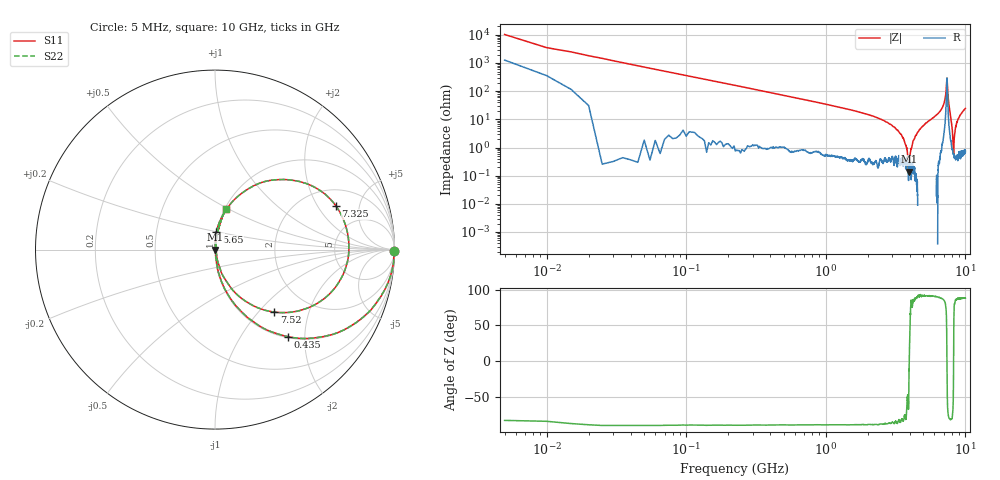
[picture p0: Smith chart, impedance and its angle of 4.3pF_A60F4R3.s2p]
! Amotech Co.,Ltd.
! http://www.amotech.co.kr/
! Part Number: A60F4R3
! These Parameters are Measured in Series Mode Connection
! Operation Temp=25[degC], DC Bias Voltage=0[V]
! Freq. Start=5[MHz] Stop=10[GHz], 2000[Steps]
! Date: Monday, July 20, 2020, 03:25:52
# GHZ S RI R 50.000000
!Freq.(Hz) S11(Real) S11(Imag) S21(Real) S21(Imag) S12(Real) S12(Imag) S22(Real) S22(Imag)
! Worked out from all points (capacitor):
!   2000 points, 5 MHz to 10 GHz, reference 50 ohm
!   read as one part in series: C = 4.43 pF near 55 MHz
!   lowest |Z| = 139 mohm at 3.935 GHz (marker M1)
!   series resonance near 3.962 GHz, so ESL is about 360 pH
!   S11 on the Smith chart (normalised r, x): 5 MHz: open; 435 MHz: 1.02, -1.65; 5.65 GHz: 1.00, +0.20; 7.325 GHz: 2.93, +2.93; 7.52 GHz: 1.35, -1.22; 10 GHz: 1.02, +0.49
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0.005  0.9987 -0.00957  0.00128 0.00957  0.00128 0.00957  0.9987 -0.00957
0.065  0.9679 -0.1757  0.0321 0.1757  0.0321 0.1757  0.9679 -0.1757
0.125  0.8905 -0.3083  0.1095 0.3083  0.1095 0.3083  0.8905 -0.3083
0.435  0.4061 -0.4849  0.5939 0.4849  0.5939 0.4849  0.4061 -0.4849
1.675  0.0382 -0.1824  0.9618 0.1824  0.9618 0.1824  0.0382 -0.1824
3.34  0.00643 -0.0353  0.9936 0.0353  0.9936 0.0353  0.00643 -0.0353
3.77  0.00239 -0.0109  0.9976 0.0109  0.9976 0.0109  0.00239 -0.0109
3.935  0.00112 -0.000825  0.9989 0.000825  0.9989 0.000825  0.00112 -0.000825
4.045  0.00235 0.00698  0.9977 -0.00698  0.9977 -0.00698  0.00235 0.00698
4.235  0.00161 0.018  0.9984 -0.018  0.9984 -0.018  0.00161 0.018
5.005  0.00288 0.0608  0.9971 -0.0608  0.9971 -0.0608  0.00288 0.0608
5.65  0.0077 0.0994  0.9923 -0.0994  0.9923 -0.0994  0.0077 0.0994
6.67  0.0497 0.2013  0.9503 -0.2013  0.9503 -0.2013  0.0497 0.2013
7.1  0.1966 0.3448  0.8034 -0.3448  0.8034 -0.3448  0.1966 0.3448
7.325  0.6733 0.2439  0.3267 -0.2439  0.3267 -0.2439  0.6733 0.2439
7.39  0.7389 -0.0624  0.2611 0.0624  0.2611 0.0624  0.7389 -0.0624
7.52  0.3305 -0.3485  0.6695 0.3485  0.6695 0.3485  0.3305 -0.3485
8.025  0.0114 -0.0507  0.9886 0.0507  0.9886 0.0507  0.0114 -0.0507
8.21  0.00571 -0.00413  0.9943 0.00413  0.9943 0.00413  0.00571 -0.00413
8.335  0.00509 0.0238  0.9949 -0.0238  0.9949 -0.0238  0.00509 0.0238
8.825  0.0137 0.0946  0.9863 -0.0946  0.9863 -0.0946  0.0137 0.0946
10  0.0634 0.2287  0.9366 -0.2287  0.9366 -0.2287  0.0634 0.2287
